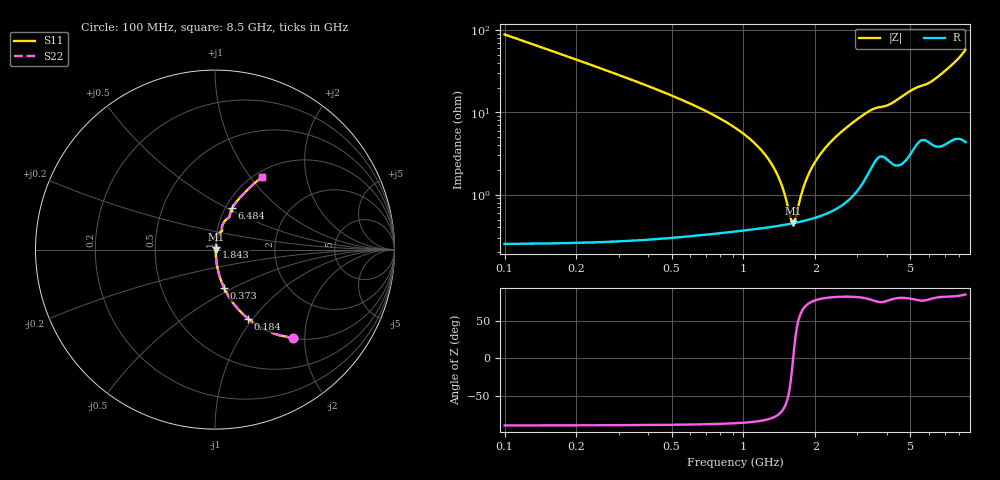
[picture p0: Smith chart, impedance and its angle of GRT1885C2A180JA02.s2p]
!Murata Part Number: GRT1885C2A180JA02
!These Parameters are Measured in Series Mode Connection
!Data Generated on Jun 19, 2026
!  o--ll--o
!Port1  Port2
!  o------o
!Operation Temp=25[degC], DC Bias Voltage=0[V]
!Freq. Start=100[MHz] Stop=9[GHz] 401[Steps]
# Hz S RI R 50
!Freq.(Hz) S11(Real) S11(Imag) S21(Real) S21(Imag) S12(Real) S12(Imag) S22(Real) S22(Imag)
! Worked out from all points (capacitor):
!   401 points, 100 MHz to 8.5 GHz, reference 50 ohm
!   read as one part in series: C = 18 pF near 142 MHz
!   lowest |Z| = 451 mohm at 1.612 GHz (marker M1)
!   series resonance near 1.615 GHz, so ESL is about 540 pH
!   S11 on the Smith chart (normalised r, x): 100 MHz: 1.01, -1.76; 184 MHz: 1.01, -0.95; 373 MHz: 1.01, -0.45; 1.843 GHz: 1.01, +0.03; 6.484 GHz: 1.08, +0.53; 8.5 GHz: 1.09, +1.14
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1e8  0.437 -0.4946  0.563 0.4946  0.563 0.4946  0.437 -0.4946
1.84e8  0.1849 -0.3855  0.8151 0.3855  0.8151 0.3855  0.1849 -0.3855
2.68e8  0.0953 -0.2894  0.9047 0.2894  0.9047 0.2894  0.0953 -0.2894
3.73e8  0.0503 -0.2125  0.9497 0.2125  0.9497 0.2125  0.0503 -0.2125
6.88e8  0.0141 -0.1035  0.9859 0.1035  0.9859 0.1035  0.0141 -0.1035
1.213e9  0.00494 -0.0319  0.9951 0.0319  0.9951 0.0319  0.00494 -0.0319
1.381e9  0.00445 -0.0174  0.9956 0.0174  0.9956 0.0174  0.00445 -0.0174
1.507e9  0.00438 -0.00769  0.9956 0.00769  0.9956 0.00769  0.00438 -0.00769
1.57e9  0.00442 -0.00314  0.9956 0.00314  0.9956 0.00314  0.00442 -0.00314
1.612e9  0.00448 -0.000209  0.9955 0.000209  0.9955 0.000209  0.00448 -0.000209
1.654e9  0.00456 0.00266  0.9954 -0.00266  0.9954 -0.00266  0.00456 0.00266
1.759e9  0.00482 0.00958  0.9952 -0.00958  0.9952 -0.00958  0.00482 0.00958
1.843e9  0.00511 0.0149  0.9949 -0.0149  0.9949 -0.0149  0.00511 0.0149
2.011e9  0.00588 0.0251  0.9941 -0.0251  0.9941 -0.0251  0.00588 0.0251
2.221e9  0.00722 0.0372  0.9928 -0.0372  0.9928 -0.0372  0.00722 0.0372
2.914e9  0.0157 0.075  0.9843 -0.075  0.9843 -0.075  0.0157 0.075
3.439e9  0.0311 0.0997  0.9689 -0.0997  0.9689 -0.0997  0.0311 0.0997
4.3e9  0.0388 0.1257  0.9612 -0.1257  0.9612 -0.1257  0.0388 0.1257
5.707e9  0.081 0.1841  0.919 -0.1841  0.919 -0.1841  0.081 0.1841
6.484e9  0.0954 0.2301  0.9046 -0.2301  0.9046 -0.2301  0.0954 0.2301
7.114e9  0.1281 0.2769  0.8719 -0.2769  0.8719 -0.2769  0.1281 0.2769
8.5e9  0.2634 0.4041  0.7366 -0.4041  0.7366 -0.4041  0.2634 0.4041
